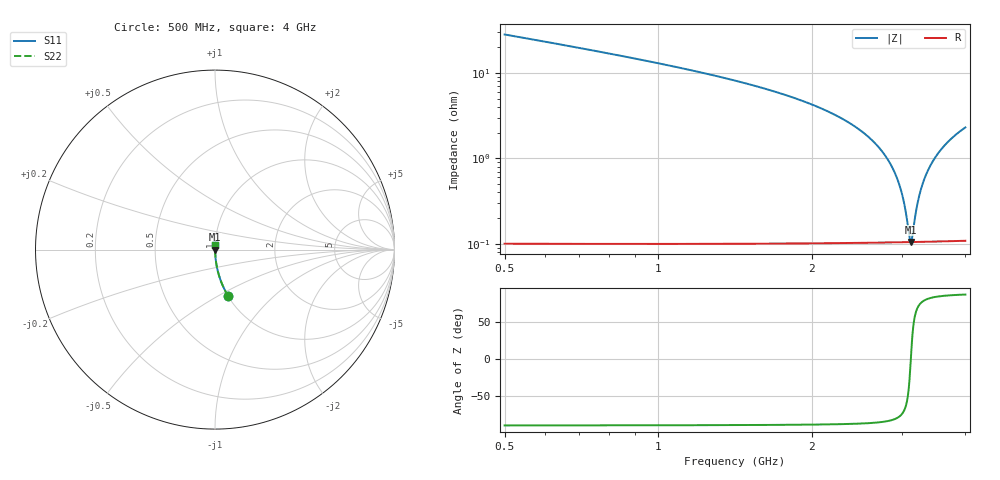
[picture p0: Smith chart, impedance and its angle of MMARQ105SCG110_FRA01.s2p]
! MMARQ105SCG110_FRA01  S-PARAMETER MODEL  ( General Type )
! Model Generated by TAIYO YUDEN Corporation (http://www.ty-top.com)
! Version 1.0
! TAIYO YUDEN Control No. 200326
! Copyright(c) 2020 TAIYO YUDEN CO.,LTD. All Rights Reserved.
! Product Description (link to TY-COMPAS)
! https://ds.yuden.co.jp/TYCOMPAS/or/detail?pn=MMARQ105SCG110JFRA01&u=M
! Products Name : Multilayer Ceramic Capacitors
! Characteristics :
!  Capacitance : 11 pF , Rated Voltage : 250V , TCC : CG / C0G
!  Case Size : 1.0 x 0.5 / 0.039 x 0.02 [mm/inch] , Thickness : 0.5 / 0.02 [mm/inch]
!  (Conditions: Temperature = 25 degC , DC Bias Current/Voltage = 0A / 0V)
! External Node Assignments :
!  1  o---| |---o  2
! GND o---------o GND
! Frequency Range : 500MHz  -  4GHz  [ 401 STEP ]
# MHz S RI R 50
! Freq[MHz].  S11 Real  S11 Imag  S21 Real  S21 Imag  S12 Real  S12 Imag  S22 Real  S22 Imag
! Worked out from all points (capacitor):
!   401 points, 500 MHz to 4 GHz, reference 50 ohm
!   read as one part in series: C = 11 pF near 517.5 MHz
!   lowest |Z| = 105 mohm at 3.125 GHz (marker M1)
!   series resonance near 3.127 GHz, so ESL is about 240 pH
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500  0.0743 -0.2604  0.9257 0.2604  0.9257 0.2604  0.0743 -0.2604
762.5  0.0317 -0.1724  0.9683 0.1724  0.9683 0.1724  0.0317 -0.1724
1086.25  0.0145 -0.1152  0.9855 0.1152  0.9855 0.1152  0.0145 -0.1152
1672.5  0.00478 -0.0613  0.9952 0.0613  0.9952 0.0613  0.00478 -0.0613
2250  0.00197 -0.0309  0.998 0.0309  0.998 0.0309  0.00197 -0.0309
2600  0.00132 -0.0171  0.9987 0.0171  0.9987 0.0171  0.00132 -0.0171
2731.25  0.00119 -0.0125  0.9988 0.0125  0.9988 0.0125  0.00119 -0.0125
2836.25  0.00112 -0.00901  0.9989 0.00901  0.9989 0.00901  0.00112 -0.00901
2923.75  0.00108 -0.0062  0.9989 0.0062  0.9989 0.0062  0.00108 -0.0062
2993.75  0.00106 -0.00402  0.9989 0.00402  0.9989 0.00402  0.00106 -0.00402
3046.25  0.00105 -0.00241  0.999 0.00241  0.999 0.00241  0.00105 -0.00241
3107.5  0.00105 -0.000578  0.999 0.000578  0.999 0.000578  0.00105 -0.000578
3125  0.00105 -6.06e-05  0.999 6.06e-05  0.999 6.06e-05  0.00105 -6.06e-05
3142.5  0.00105 0.000454  0.999 -0.000454  0.999 -0.000454  0.00105 0.000454
3212.5  0.00105 0.00249  0.9989 -0.00249  0.9989 -0.00249  0.00105 0.00249
3265  0.00107 0.00398  0.9989 -0.00398  0.9989 -0.00398  0.00107 0.00398
3335  0.00109 0.00594  0.9989 -0.00594  0.9989 -0.00594  0.00109 0.00594
3422.5  0.00113 0.00833  0.9989 -0.00833  0.9989 -0.00833  0.00113 0.00833
3527.5  0.00119 0.0111  0.9988 -0.0111  0.9988 -0.0111  0.00119 0.0111
3658.75  0.00128 0.0145  0.9987 -0.0145  0.9987 -0.0145  0.00128 0.0145
3825  0.00142 0.0187  0.9986 -0.0187  0.9986 -0.0187  0.00142 0.0187
4000  0.00161 0.0229  0.9984 -0.0229  0.9984 -0.0229  0.00161 0.0229
